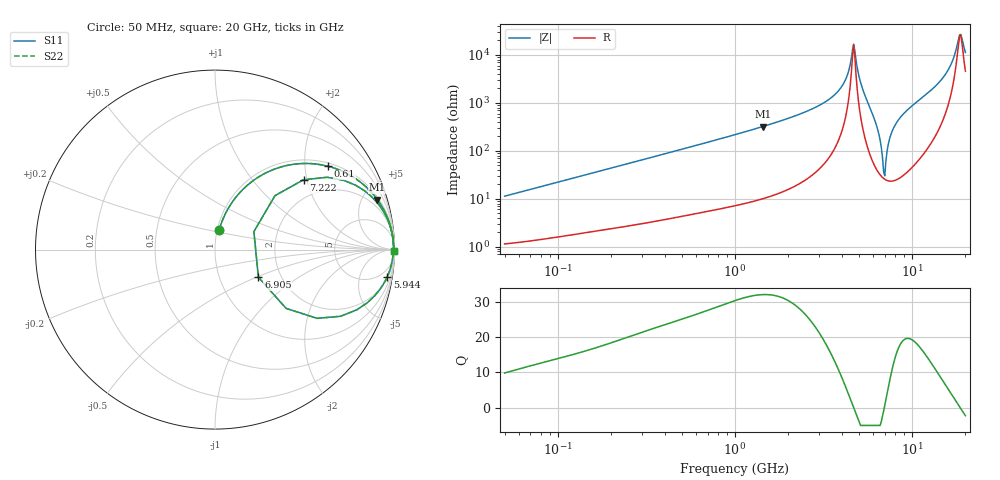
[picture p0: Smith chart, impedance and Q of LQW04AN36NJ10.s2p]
!Murata Part Number: LQW04AN36NJ10
!These Parameters are Measured in Series Mode Connection
!  o--[Z]--o
!Port1  Port2
!  o-------o
!Freq. Start=50[MHz] Stop=20[GHz], 401[Steps]
# Hz S RI R 50
!Freq.(Hz) S11(Real) S11(Imag) S21(Real) S21(Imag) S12(Real) S12(Imag) S22(Real) S22(Imag)
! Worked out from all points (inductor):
!   401 points, 50 MHz to 20 GHz, reference 50 ohm
!   read as one part in series: L = 35.8 nH near 51.52 MHz
!   highest Q = 32 at 1.433 GHz (marker M1), where L = 35.6 nH
!   self-resonance near 4.678 GHz
!   S11 on the Smith chart (normalised r, x): 50 MHz: 1.02, +0.23; 610 MHz: 1.10, +2.63; 5.944 GHz: 2, -12; 6.905 GHz: 1.53, -0.51; 7.222 GHz: 1.48, +1.91; 20 GHz: open
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5e7  0.0236 0.1091  0.9764 -0.1091  0.9764 -0.1091  0.0236 0.1091
1.364002e8  0.0977 0.2669  0.9023 -0.2669  0.9023 -0.2669  0.0977 0.2669
3.721004e8  0.3981 0.4682  0.6019 -0.4682  0.6019 -0.4682  0.3981 0.4682
6.100003e8  0.6293 0.4645  0.3707 -0.4645  0.3707 -0.4645  0.6293 0.4645
1e9  0.818 0.3697  0.182 -0.3697  0.182 -0.3697  0.818 0.3697
1.432596e9  0.9043 0.2789  0.0957 -0.2789  0.0957 -0.2789  0.9043 0.2789
2.728004e9  0.9774 0.1294  0.0226 -0.1294  0.0226 -0.1294  0.9774 0.1294
3.908127e9  0.9922 0.0508  0.00777 -0.0508  0.00777 -0.0508  0.9922 0.0508
4.275624e9  0.9938 0.0276  0.00619 -0.0276  0.00619 -0.0276  0.9938 0.0276
4.677679e9  0.994 0.000131  0.00599 -0.000131  0.00599 -0.000131  0.994 0.000131
5.194772e9  0.9905 -0.0435  0.00952 0.0435  0.00952 0.0435  0.9905 -0.0435
5.944466e9  0.9591 -0.1526  0.0409 0.1526  0.0409 0.1526  0.9591 -0.1526
6.311513e9  0.8886 -0.2587  0.1114 0.2587  0.1114 0.2587  0.8886 -0.2587
6.601595e9  0.7004 -0.3714  0.2996 0.3714  0.2996 0.3714  0.7004 -0.3714
6.905011e9  0.2417 -0.154  0.7583 0.154  0.7583 0.154  0.2417 -0.154
7.222371e9  0.4932 0.389  0.5068 -0.389  0.5068 -0.389  0.4932 0.389
7.442007e9  0.7202 0.3851  0.2798 -0.3851  0.2798 -0.3851  0.7202 0.3851
8.516016e9  0.9483 0.1948  0.0517 -0.1948  0.0517 -0.1948  0.9483 0.1948
1.527346e10  0.9954 0.0262  0.00455 -0.0262  0.00455 -0.0262  0.9954 0.0262
1.670968e10  0.9961 0.0142  0.00395 -0.0142  0.00395 -0.0142  0.9961 0.0142
1.855685e10  0.9963 0.00102  0.00365 -0.00102  0.00365 -0.00102  0.9963 0.00102
2e10  0.9963 -0.00805  0.00367 0.00805  0.00367 0.00805  0.9963 -0.00805
